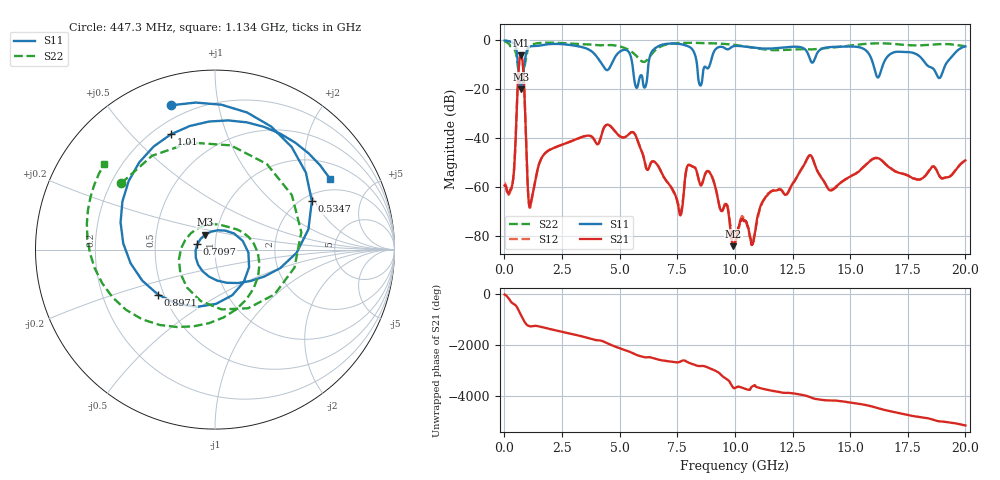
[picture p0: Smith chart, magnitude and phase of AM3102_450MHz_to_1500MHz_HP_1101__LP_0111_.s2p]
!Agilent Technologies,E8364B,MY43040894,A.07.50.67
!Agilent E8364B: A.07.50.67
!Date: Thursday, January 11, 2018 06:39:05
!Correction: S11(Full 2 Port(1,2))
!S21(Full 2 Port(1,2))
!S12(Full 2 Port(1,2))
!S22(Full 2 Port(1,2))
!S2P File: Measurements: S11, S21, S12, S22:
# Hz S  dB  R 50
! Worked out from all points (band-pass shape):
!   1601 points, 10 MHz to 20 GHz, reference 50 ohm
!   highest |S21| = -6.18 dB at 709.6 MHz (marker M1); lowest = -84.4 dB at 9.93 GHz (marker M2)
!   |S21| within 3 dB of the highest: 642.3 MHz to 793.9 MHz (151.6 MHz wide, 21.1 % of centre)
!   lowest |S11| = -20.0 dB at 734.6 MHz (marker M3), VSWR 1.22, Z = 44.3 + j7.49 ohm
!   |S11| at or under -10 dB: 5.555 GHz to 6.246 GHz (690.6 MHz wide, 11.7 % of centre); 8.357 GHz to 8.916 GHz (559.2 MHz wide, 6.48 % of centre); 18.32 GHz to 19.14 GHz (818.7 MHz wide, 4.37 % of centre)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
!   |S22| runs from -17.0 to -0.4 dB; largest |S21 - S12| = 0.00068
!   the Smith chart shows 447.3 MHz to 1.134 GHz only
!   S11 on the Smith chart (normalised r, x): 447.3 MHz: 0.13, +0.73; 534.7 MHz: 2.23, +1.90; 709.6 MHz: 0.82, +0.05; 897.1 MHz: 0.47, -0.28; 1.01 GHz: 0.27, +0.66; 1.134 GHz: 1.52, +2.77
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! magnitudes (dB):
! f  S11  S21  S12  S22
! 10 MHz  -0.1  -59.5  -58.5  -0.4
! 447.3 MHz  -1.5  -48.8  -48.9  -3.9
! 534.7 MHz  -4.4  -28.2  -28.2  -6.9
! 709.6 MHz  -19.7  -6.2  -6.2  -16.9
! 734.6 MHz  -20.0  -6.4  -6.4  -17.0
! 897.1 MHz  -7.9  -28.5  -28.6  -9.7
! 1.01 GHz  -3.2  -59.0  -59.4  -4.0
! 1.134 GHz  -2.5  -67.6  -67.8  -2.2
! 1.722 GHz  -1.8  -46.7  -46.8  -1.0
! 3.346 GHz  -2.7  -39.7  -39.7  -1.6
! 5.32 GHz  -4.1  -39.2  -39.2  -3.6
! 5.745 GHz  -19.5  -40.2  -40.2  -6.6
! 6.682 GHz  -2.4  -51.7  -51.6  -3.1
! 7.631 GHz  -1.5  -71.8  -70.1  -1.1
! 7.981 GHz  -2.5  -51.1  -51.0  -1.0
! 8.881 GHz  -10.9  -53.9  -53.9  -1.2
! 9.93 GHz  -2.4  -84.4  -81.1  -1.8
! 10.01 GHz  -2.3  -83.0  -82.6  -1.9
! 13.34 GHz  -9.1  -47.7  -47.8  -3.7
! 14.15 GHz  -2.8  -61.5  -61.3  -3.1
! 16.68 GHz  -6.1  -51.9  -51.7  -1.3
! 20 GHz  -2.5  -49.2  -49.4  -2.4
